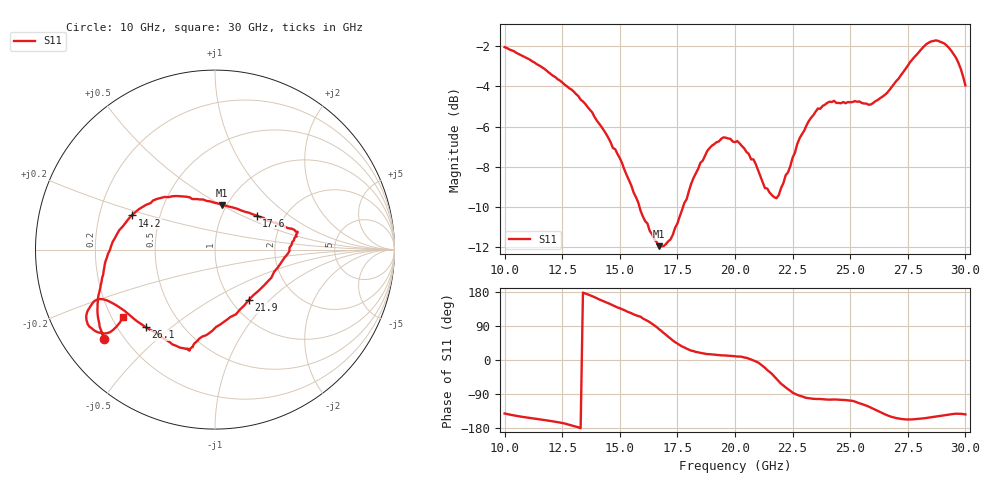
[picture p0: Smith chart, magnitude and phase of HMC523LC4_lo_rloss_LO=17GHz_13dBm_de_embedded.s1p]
!Hittite Microwave Corporation
!20 Alpha Rd
!Chelmsford, MA 01824
!Tel: 978-250-3343
!Fax: 978-250-3373
!Device: HMC523LC4, 10-30 GHz, GaAs MMIC Double-Balanced Mixer
!Misc: LO Return Loss with LO at 13 dBm, Room
# MHZ S MA R 50
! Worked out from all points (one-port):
!   201 points, 10 GHz to 30 GHz, reference 50 ohm
!   lowest |S11| = -12.0 dB at 16.7 GHz (marker M1), VSWR 1.67, Z = 47.3 + j25.2 ohm
!   |S11| at or under -10 dB: 15.85 GHz to 17.75 GHz (1.897 GHz wide, 11.3 % of centre)
!   S11 on the Smith chart (normalised r, x): 10 GHz: 0.13, -0.35; 14.2 GHz: 0.34, +0.17; 17.6 GHz: 1.45, +0.60; 21.9 GHz: 1.20, -0.76; 26.1 GHz: 0.31, -0.41; 30 GHz: 0.25, -0.31
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10000  0.791 -141.1
11000  0.741 -152.1
12500  0.646 -166.3
13500  0.571 175.5
14200  0.501 157.7
15000  0.418 136.6
15700  0.334 118.2
16700  0.252 81.5
17500  0.287 43.4
17600  0.299 39.3
18800  0.436 15.5
19500  0.471 12.2
20000  0.458 9.9
20500  0.433 5.8
20900  0.404 -3.7
21300  0.352 -20.6
21900  0.338 -56.3
22500  0.419 -86.1
23300  0.527 -101.7
24100  0.578 -104.7
25000  0.576 -107.1
26100  0.58 -131.9
26800  0.629 -150.2
27500  0.711 -157.0
28200  0.794 -153.9
28700  0.822 -149.7
29500  0.758 -142.2
30000  0.635 -143.7
